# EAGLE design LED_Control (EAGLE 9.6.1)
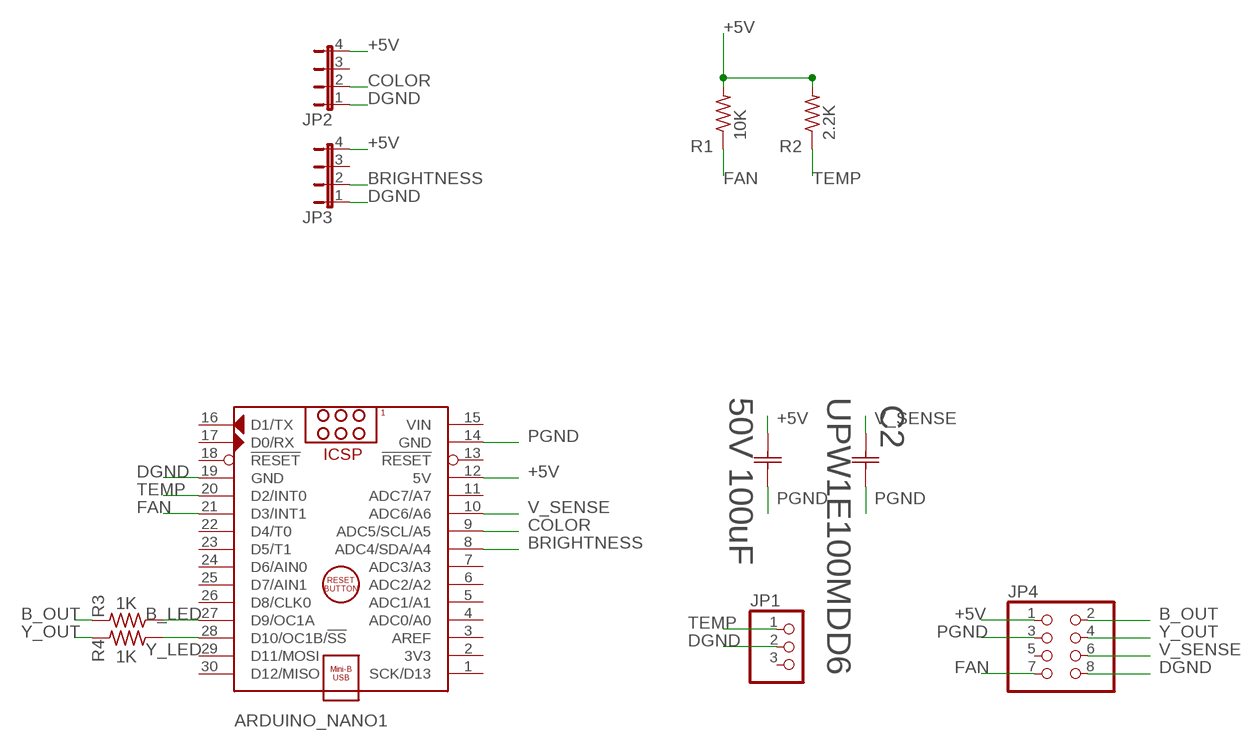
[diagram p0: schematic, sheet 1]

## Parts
ARDUINO_NANO1  ARDUINO_NANO  [ARDUINO_NANO]
C1  50YXJ100MT78X11.5  [CAP_YX_8X11P5_RUB]
C2  UPW1E100MDD6  [U1-A_NCH]
JP1  PINHD-1X3  [1X03]
JP2  JP4E  [JP4]
JP3  JP4E  [JP4]
JP4  PINHD-2X4  [2X04]
R1  10K  R-US_0207/10  [0207/10]
R2  2.2K  R-US_0207/10  [0207/10]
R3  1K  R-US_0207/10  [0207/10]
R4  1K  R-US_0207/10  [0207/10]

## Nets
+5V [Power]: ARDUINO_NANO1.12(5V) C1.1 JP2.4 JP3.4 JP4.1 R1.2 R2.2
B_LED [Data]: ARDUINO_NANO1.27(D9/OC1A) R3.1
B_OUT: JP4.2 R3.2
BRIGHTNESS [Data]: ARDUINO_NANO1.8(ADC4/SDA/A4) JP3.2
COLOR [Data]: ARDUINO_NANO1.9(ADC5/SCL/A5) JP2.2
DGND [Power]: ARDUINO_NANO1.19(GND) JP1.2 JP2.1 JP3.1 JP4.8
FAN [Data]: ARDUINO_NANO1.21(D3/INT1) JP4.7 R1.1
PGND [Power]: ARDUINO_NANO1.14(GND) C1.2 C2.2 JP4.3
TEMP [Data]: ARDUINO_NANO1.20(D2/INT0) JP1.1 R2.1
V_SENSE [Data]: ARDUINO_NANO1.10(ADC6/A6) C2.1 JP4.6
Y_LED [Data]: ARDUINO_NANO1.28(D10/OC1B/!SS) R4.1
Y_OUT: JP4.4 R4.2
Unconnected: ARDUINO_NANO1.1(SCK/D13) ARDUINO_NANO1.2(3V3) ARDUINO_NANO1.3(AREF) ARDUINO_NANO1.4(ADC0/A0) ARDUINO_NANO1.5(ADC1/A1) ARDUINO_NANO1.6(ADC2/A2) ARDUINO_NANO1.7(ADC3/A3) ARDUINO_NANO1.11(ADC7/A7) ARDUINO_NANO1.13(!RESET) ARDUINO_NANO1.16(D1/TX) ARDUINO_NANO1.17(D0/RX) ARDUINO_NANO1.18(!RESET) ARDUINO_NANO1.22(D4/T0) ARDUINO_NANO1.23(D5/T1) ARDUINO_NANO1.24(D6/AIN0) ARDUINO_NANO1.25(D7/AIN1) ARDUINO_NANO1.26(D8/CLK0) ARDUINO_NANO1.29(D11/MOSI) ARDUINO_NANO1.30(D12/MISO) JP1.3 JP2.3 JP3.3 JP4.5

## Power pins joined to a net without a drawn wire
VIN: ARDUINO_NANO1.15(VIN)

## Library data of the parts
ARDUINO_NANO1 = ArduinoNanoV30:ARDUINO_NANO: Arduino Nano V3.0 Module Overview: The Arduino Nano is a small, complete, and breadboard-friendly board based on the ATmega328 (Arduino Nano 3.x) or ATmega168 (Arduino Nano 2.x). It has more or less the same functionality of the Arduino Duemilanove, but in a different package. It lacks only a DC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
C1 = Added Capacitors:50YXJ100MT78X11.5: CAP ALUM 100UF 20% 50V RADIAL; BUILT_BY: EMA_Cory; COPYRIGHT: Copyright (C) 2018 Accelerated Designs. All rights reserved; MANUFACTURER_PART_NUMBER: 50YXJ100MT78X11.5; SOURCELIBRARY: Rubycon_2019-09-19; VENDOR: Rubycon Netherlands
C2 = Digikey Components:UPW1E100MDD6: UPW1E100MDD6 10uF 25V Electrolytic Capacitor; BUILT_BY: EMA_UL_Team; MANUFACTURER_PART_NUMBER: UPW1E100MDD6; SOURCELIBRARY: Nichicon_2014-12-31; VENDOR: Nichicon
JP1 = Silent_Headers:PINHD-1X3: PIN HEADER
JP2 JP3 = Jumper_Silent:JP4E: JUMPER
JP4 = Silent_Headers:PINHD-2X4: PIN HEADER
R1-R4 = rcl:R-US_: RESISTOR, American symbol; SPICEPREFIX: R

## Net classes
1 Data: width 0.254 mm
2 Power: width 0.508 mm

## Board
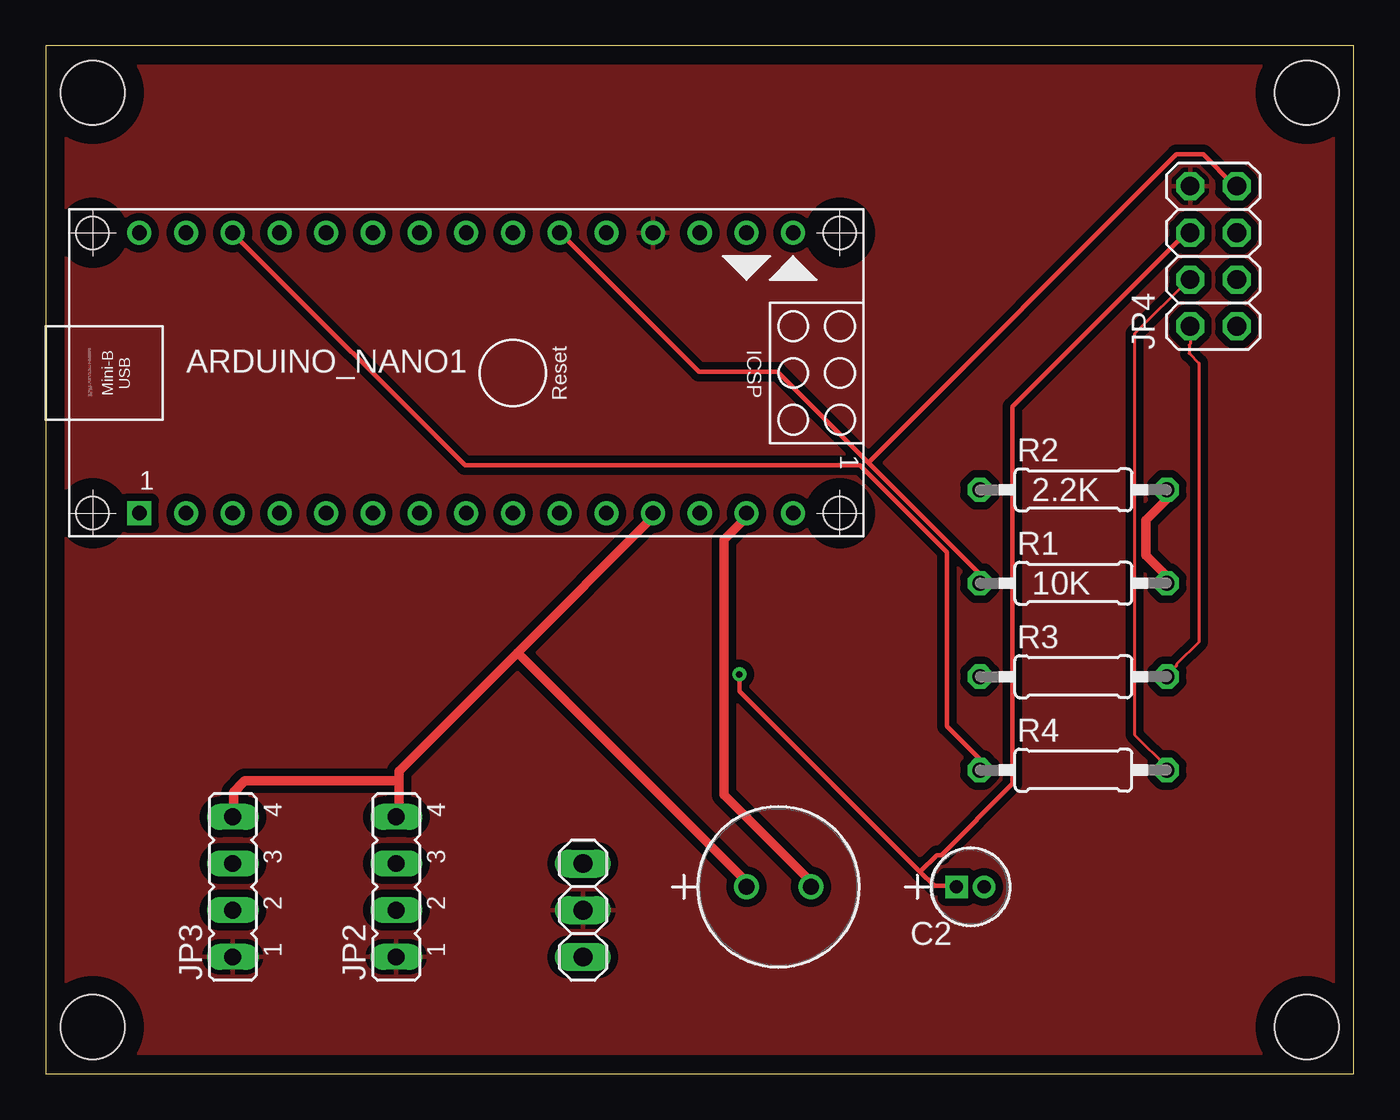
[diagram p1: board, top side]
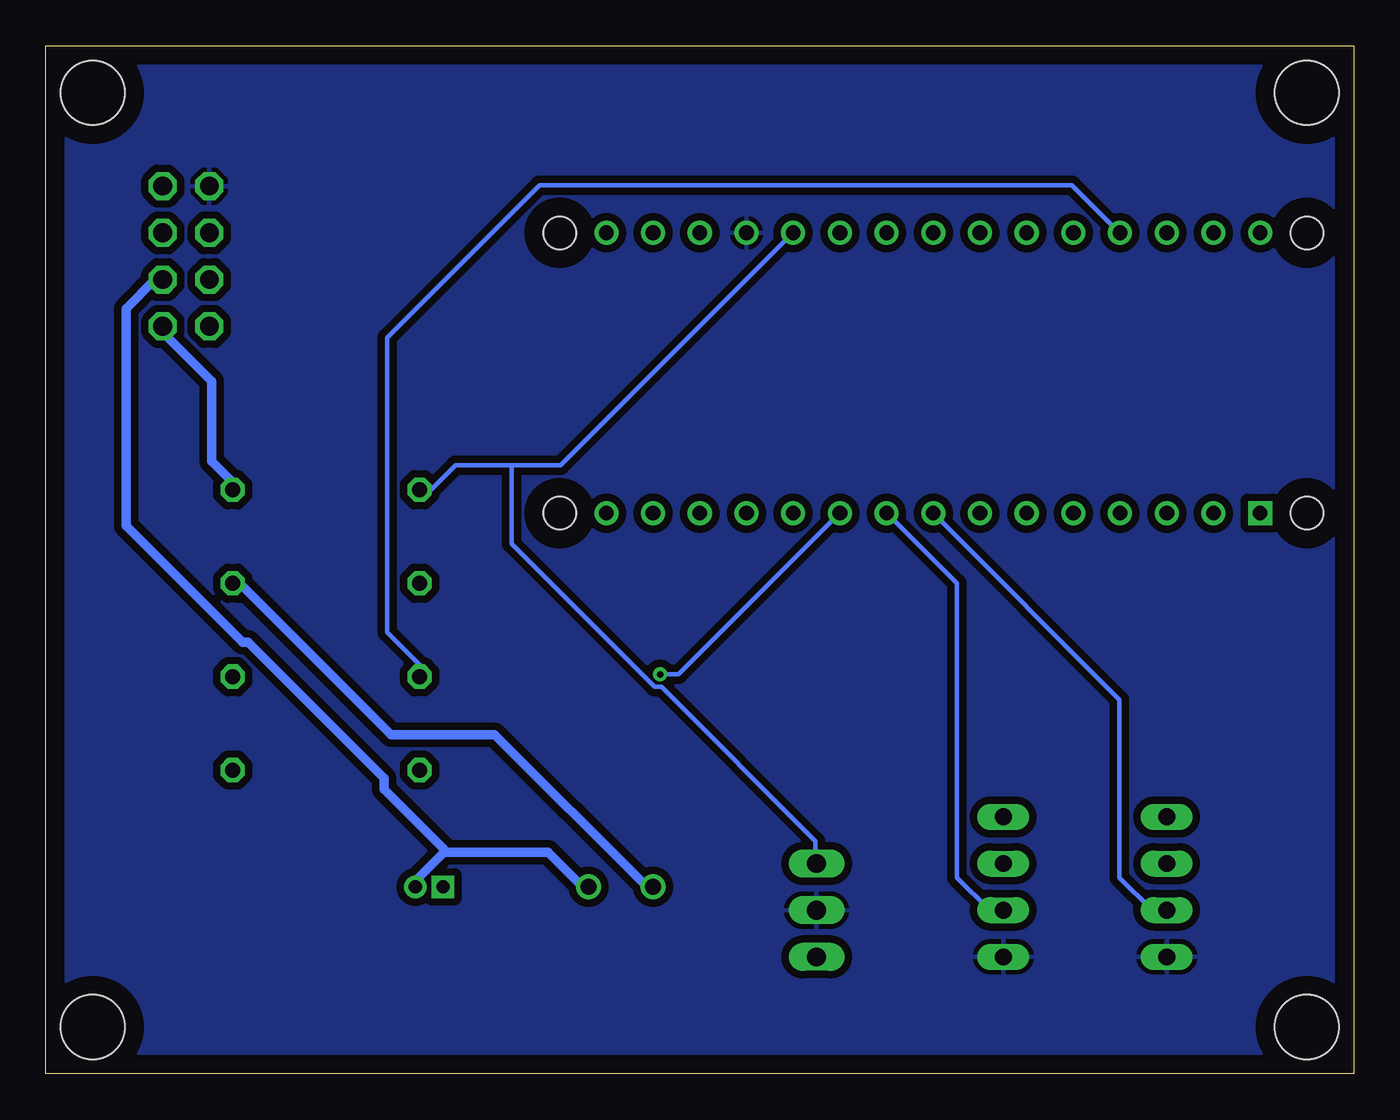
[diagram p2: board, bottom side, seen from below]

Size 71.12 x 55.88 mm. Coordinates in mm from the lower left corner, seen from the top.
Outline: 0,0 71.12,0 71.12,55.88 0,55.88 0,0
Copper layers (1*16): Top 0.035mm / dielectric 1.5mm / Bottom 0.035mm
Design rules "default": minimum track width 6mil, minimum drill 0.35mm, track to track 6mil, track to pad 6mil, pad to pad 6mil, via to via 6mil, smd to smd 6mil, copper to edge 40mil, drill to drill 6mil, minimum pad ring 10mil, minimum via ring 8mil, stop-mask expansion 4mil, vias tented up to drill 0mil, thermal gap 10mil
Holes 3.5 mm at 2.54,53.34 68.58,53.34 68.58,2.54 2.54,2.54

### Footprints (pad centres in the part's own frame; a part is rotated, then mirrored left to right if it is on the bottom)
ARDUINO_NANO = drill 0.8 square: 1 -20.32,-7.62 | drill 0.8: 2 -17.78,-7.62; 3 -15.24,-7.62; 4 -12.7,-7.62; 5 -10.16,-7.62; 6 -7.62,-7.62; 7 -5.08,-7.62; 8 -2.54,-7.62; 9 0,-7.62; 10 2.54,-7.62; 11 5.08,-7.62; 12 7.62,-7.62; 13 10.16,-7.62; 14 12.7,-7.62; 15 15.24,-7.62; 16 15.24,7.62; 17 12.7,7.62; 18 10.16,7.62; 19 7.62,7.62; 20 5.08,7.62; 21 2.54,7.62; 22 0,7.62; 23 -2.54,7.62; 24 -5.08,7.62; 25 -7.62,7.62; 26 -10.16,7.62; 27 -12.7,7.62; 28 -15.24,7.62; 29 -17.78,7.62; 30 -20.32,7.62 | hole 1.778: -22.86,-7.62; -22.86,7.62; 17.78,7.62; 17.78,-7.62
CAP_YX_8X11P5_RUB = drill 0.864 pad 1.372: 1 0,0; 2 3.505,0
U1-A_NCH = drill 0.711 pad 1.219 square: 1 0,0 | drill 0.711 pad 1.219: 2 1.499,0
1X03 = drill 1.016 long: 1 -2.54,0; 2 0,0; 3 2.54,0
JP4 = drill 0.914 long: 1 -3.81,0; 2 -1.27,0; 3 1.27,0; 4 3.81,0
2X04 = drill 1.016 octagon: 1 -3.81,-1.27; 2 -3.81,1.27; 3 -1.27,-1.27; 4 -1.27,1.27; 5 1.27,-1.27; 6 1.27,1.27; 7 3.81,-1.27; 8 3.81,1.27
0207/10 = drill 0.813 octagon: 1 -5.08,0; 2 5.08,0

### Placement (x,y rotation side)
ARDUINO_NANO1  25.4,38.1 0 top
C1  38.1,10.16 0 top
C2  49.53,10.16 0 top
JP1  29.21,8.89 270 top
JP2  19.05,10.16 90 top
JP3  10.16,10.16 90 top
JP4  63.5,44.45 90 top
R1  55.88,26.67 0 top
R2  55.88,31.75 0 top
R3  55.88,21.59 0 top
R4  55.88,16.51 0 top

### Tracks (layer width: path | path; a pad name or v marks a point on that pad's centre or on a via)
+5V
  Top 0.508: R1.2 60.96,27.05 59.82,28.19 59.82,30.1 61.04,31.32 61.04,31.62 60.96,31.7 R2.2 | 25.64,22.9 19.2,16.46 19.2,15.93 | 25.64,22.9 32.99,30.25 32.99,30.48 ARDUINO_NANO1.12 | 19.2,15.93 19.2,14.17 19.05,14.02 JP2.4 | C1.1 38.1,10.44 25.64,22.9 | 19.2,15.93 10.82,15.93 10.21,15.32 10.21,14.02 JP3.4
  Bottom 0.508: JP4.1 64.77,40.31 62.1,37.64 62.1,33.3 60.96,32.16 R2.2 | R1.2 60.58,26.67 52.35,18.44 46.71,18.44 38.48,10.21 38.1,10.21 C1.1
B_LED
  Bottom 0.254: ARDUINO_NANO1.27 12.72,45.72 15.32,48.31 44.27,48.31 52.58,40.01 52.58,24 50.75,22.17 50.75,21.64 R3.1
B_OUT
  Top 0.152: R3.2 60.96,21.64 61.49,22.17 61.49,22.25 62.71,23.47 62.71,38.63 62.18,39.17 62.18,39.62 62.26,39.7 62.26,40.62 JP4.2
BRIGHTNESS
  Bottom 0.254: ARDUINO_NANO1.8 12.72,20.34 12.72,10.67 10.97,8.91 10.21,8.91 JP3.2
COLOR
  Bottom 0.254: ARDUINO_NANO1.9 25.38,30.48 21.57,26.67 21.57,10.67 19.81,8.91 19.05,8.91 JP2.2
DGND
  pour Top (isolate 0.406): 0,55.88 0,0 71.12,0 71.12,55.88
  pour Bottom (isolate 0.406): 0,55.88 0,0 71.12,0 71.12,55.88
FAN
  Top 0.254: 44.73,33.22 50.75,27.2 50.75,26.67 R1.1 | 44.73,33.22 39.78,38.18 35.51,38.18 27.96,45.72 ARDUINO_NANO1.21 | 44.73,33.22 61.49,49.99 62.94,49.99 64.62,48.31 64.77,48.31 JP4.7
PGND
  Top 0.508: ARDUINO_NANO1.14 38.1,30.25 36.88,29.03 36.88,15.16 41.6,10.44 C1.2
  Bottom 0.508: 49.45,12.04 50.98,10.52 50.98,10.21 C2.2 | 49.45,12.04 43.81,12.04 41.99,10.21 41.6,10.21 C1.2 | JP4.3 64.77,43.13 65.23,43.13 66.75,41.6 66.75,29.79 60.43,23.47 60.12,23.47 52.73,16.08 52.73,15.47 49.53,12.27 49.45,12.04
TEMP
  Bottom 0.254: ARDUINO_NANO1.20 43.13,33.07 45.8,33.07 | 45.8,33.07 48.84,33.07 50.22,31.7 50.75,31.7 R2.1 | 45.8,33.07 45.8,28.8 38.02,21.03 37.64,21.03 29.26,12.65 29.26,11.43 JP1.1
V_SENSE  (via drill 0.35)
  Top 0.254: 47.55,10.97 37.72,20.8 v37.72,21.72 | 47.55,10.97 48.31,10.21 49.53,10.21 C2.1 | JP4.6 62.03,45.72 52.58,36.27 52.58,15.77 48.69,11.89 48.46,11.89 47.55,10.97
  Bottom 0.254: v37.72,21.72 36.73,21.72 27.96,30.48 ARDUINO_NANO1.10
Y_LED
  Top 0.254: ARDUINO_NANO1.28 10.21,45.72 10.52,45.41 10.52,45.34 22.78,33.07 44.27,33.07 49,28.35 49,18.9 50.83,17.07 50.83,16.54 R4.1
Y_OUT
  Top 0.152: R4.2 60.96,16.69 59.21,18.44 59.21,40.23 62.18,43.2 JP4.4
